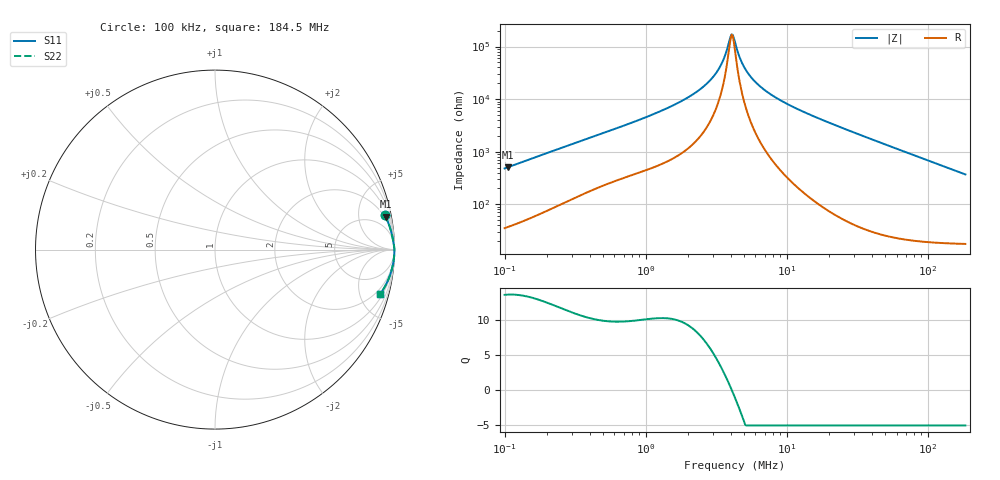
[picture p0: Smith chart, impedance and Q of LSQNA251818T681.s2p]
! LSQNA251818T681  S-PARAMETER MODEL  ( General Type )
! Model Generated by TAIYO YUDEN Corporation (http://www.ty-top.com)
! Version 2.0
! TAIYO YUDEN Control No. 100810NF25SB-FKC
! Copyright(c) 2007 TAIYO YUDEN CO.,LTD. All Rights Reserved.
! Product Description (link to TY-COMPAS)
! https://ds.yuden.co.jp/TYCOMPAS/or/detail?pn=LSQNA251818T681K&u=M
! Products Name : Inductors
! Characteristics :
!  Inductance : 680 uH , SRF(min) : 3.0 MHz , DC Resistance(max) : 22.1 Ohm
!  Rated Current : Saturation :30 mA , Temp Rise : 90 mA (40 degC)
!  Case Size : 2.5 x 1.8 / 0.098 x 0.071 [mm/inch] , Thickness : 1.8 / 0.071 [mm/inch]
!  (Conditions: Temperature = 25 degC , DC Bias Current/Voltage = 0A / 0V)
! External Node Assignments :
!  1  o---GGG---o  2
! GND o---------o GND
! Frequency Range : 0.1MHz  -  184.468258MHz  [ 402 STEP ]
# MHz S RI R 50
! Freq[MHz].  S11 Real  S11 Imag  S21 Real  S21 Imag  S12 Real  S12 Imag  S22 Real  S22 Imag
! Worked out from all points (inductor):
!   401 points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, 100 kHz to 184.5 MHz, reference 50 ohm
!   read as one part in series: L = 757 uH near 103.8 kHz
!   highest Q = 13.7 at 105.8 kHz (marker M1), where L = 761 uH
!   self-resonance near 4.059 MHz
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0.1  0.9454 0.1934  0.0546 -0.1934  0.0546 -0.1934  0.9454 0.1934
0.105802  0.9502 0.1841  0.0498 -0.1841  0.0498 -0.1841  0.9502 0.1841
0.352405  0.9906 0.0604  0.00942 -0.0604  0.00942 -0.0604  0.9906 0.0604
1.241892  0.998 0.0173  0.00198 -0.0173  0.00198 -0.0173  0.998 0.0173
1.95002  0.9989 0.00955  0.0011 -0.00955  0.0011 -0.00955  0.9989 0.00955
2.68436  0.9992 0.00514  0.000784 -0.00514  0.000784 -0.00514  0.9992 0.00514
3.061924  0.9993 0.00348  0.0007 -0.00348  0.0007 -0.00348  0.9993 0.00348
3.363709  0.9993 0.00233  0.000653 -0.00233  0.000653 -0.00233  0.9993 0.00233
3.626416  0.9994 0.00142  0.000621 -0.00142  0.000621 -0.00142  0.9994 0.00142
3.983837  0.9994 0.0003  0.00059 -0.0003  0.00059 -0.0003  0.9994 0.0003
4.136483  0.9994 -0.000149  0.000579 0.000149  0.000579 0.000149  0.9994 -0.000149
4.294977  0.9994 -0.000598  0.00057 0.000598  0.00057 0.000598  0.9994 -0.000598
4.630416  0.9994 -0.0015  0.000555 0.0015  0.000555 0.0015  0.9994 -0.0015
4.992054  0.9995 -0.00241  0.000544 0.00241  0.000544 0.00241  0.9995 -0.00241
5.484074  0.9995 -0.00358  0.000536 0.00358  0.000536 0.00358  0.9995 -0.00358
6.138922  0.9995 -0.00501  0.000534 0.00501  0.000534 0.00501  0.9995 -0.00501
7.135272  0.9995 -0.00703  0.000546 0.00703  0.000546 0.00703  0.9995 -0.00703
8.77452  0.9994 -0.0101  0.00059 0.0101  0.00059 0.0101  0.9994 -0.0101
15.13571  0.9991 -0.0206  0.000946 0.0206  0.000946 0.0206  0.9991 -0.0206
53.33896  0.9925 -0.0772  0.00748 0.0772  0.00748 0.0772  0.9925 -0.0772
99.19348  0.9755 -0.1413  0.0245 0.1413  0.0245 0.1413  0.9755 -0.1413
184.4683  0.9216 -0.2461  0.0784 0.2461  0.0784 0.2461  0.9216 -0.2461
